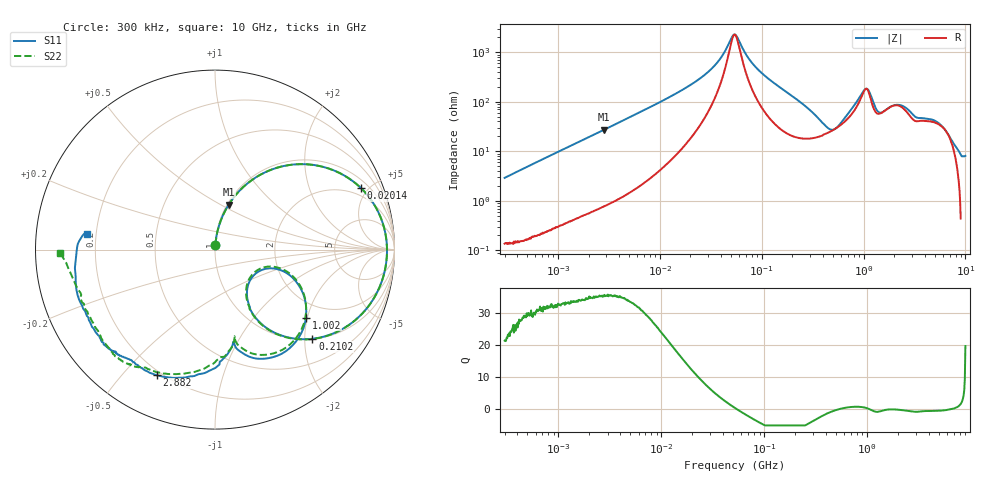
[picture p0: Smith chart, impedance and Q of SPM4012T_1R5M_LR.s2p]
! S-Parameter Data Generated by TDK Corporation
! Copyright(C) 2019 TDK Corporation.
! All Rights Reserved.
! TDK P/N: SPM4012T-1R5M-LR (Inductor)
! Property: L=1.5uH at 100kHz
! Size(LxWxT): 4.4x4.1x1.2mm
! Model Type: s2p (Touchstone File Format Version 1.0)
! Frequency: DC=Yes Start=0.3MHz Stop=10000MHz 802points Log-sweep
! Model Generated on Sep. 23, 2019
! Port Assignments:
!  1 ---@@@--- 2
! Applicable Conditions:
!  Temperature = 25 degC
!  DC Bias Current = 0 A
!  Small Signal Operation
! Terms and conditions regarding TDK Simulation Models
! (1)This simulation model is being provided solely for informational purposes. Please refer to the specifications of the products in terms of detailed characteristics of such products.
! (2)In no event shall TDK Corporation of any of its subsidiaries be liable for any loss or damage arising, directly or indirectly,
!  From any information contained in this simulation model, including, but not limited to loss or damages arising from any inaccuracies, omissions or errors in connection with such information.
! (3)Any and all copyrights on this simulation model are owned by TDK Corporation.
!  Duplication or redistribution of this simulation model without prior written permission from TDK Corporation is prohibited.
! (4)This simulation model is subject to any modification or change without any prior notice.
! (5)Neither TDK Corporation nor any of its subsidiaries shall make any warranty, express or implied,
!  Including but not limited to the correctness, implied warranties of merchantability and fitness for a particular purpose with respect to this simulation models.
! (6)The use of this simulation model shall be deemed to have consented to the terms and conditions hereof.
# Hz S MA R 50
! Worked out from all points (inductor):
!   801 points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, 300 kHz to 10 GHz, reference 50 ohm
!   read as one part in series: L = 1.55 uH near 318.3 kHz
!   highest Q = 35.3 at 2.857 MHz (marker M1), where L = 1.53 uH
!   self-resonance near 54.41 MHz
!   S11 on the Smith chart (normalised r, x): 300 kHz: 1.00, +0.06; 20.14 MHz: 1.45, +4.51; 210.2 MHz: 1.01, -2.18; 1.002 GHz: 1.55, -1.96; 2.882 GHz: 0.18, -0.62; 10 GHz: 0.17, +0.06
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300000  0.02814 85.6  0.9981 -1.7  0.9984 -1.7  0.02796 85.3
1713600  0.1618 78.9  0.9821 -9.4  0.9821 -9.4  0.1617 78.9
2857356  0.2617 73.1  0.9577 -15.3  0.9578 -15.3  0.2617 73.1
9671944  0.6725 45.1  0.713 -42.6  0.7131 -42.6  0.6724 45.1
2.013744e7  0.8828 22.8  0.4015 -62.4  0.4016 -62.4  0.8828 22.8
3.467969e7  0.9473 8.5  0.1749 -68.9  0.1749 -68.9  0.9473 8.5
5.477226e7  0.958 -2.2  0.04202 1.1  0.04203 1.1  0.9581 -2.3
9.327145e7  0.9317 -15.4  0.2115 61.8  0.2116 61.8  0.9317 -15.5
2.102074e8  0.7359 -42.5  0.5739 38.6  0.574 38.6  0.735 -42.7
3.126428e8  0.5295 -56.4  0.7247 18.8  0.7248 18.8  0.5275 -56.7
4.20949e8  0.3507 -58.0  0.7739 1.6  0.774 1.6  0.3465 -58.4
5.663179e8  0.2583 -35.1  0.7495 -17.1  0.7495 -17.1  0.2495 -34.7
7.84152e8  0.4135 -18.0  0.5965 -38.6  0.5965 -38.6  0.4051 -16.5
1.001841e9  0.6328 -36.8  0.3544 -42.8  0.3544 -42.8  0.6204 -35.3
1.180962e9  0.6802 -61.9  0.3702 -15.5  0.3702 -15.5  0.6638 -60.5
1.35547e9  0.5752 -76.9  0.4999 -23.4  0.5 -23.4  0.555 -75.8
1.767019e9  0.5623 -81.1  0.4464 -46.3  0.4464 -46.4  0.5286 -78.8
2.882439e9  0.772 -114.9  0.3385 -51.9  0.3385 -51.9  0.7493 -112.8
4.749267e9  0.8017 -135.3  0.2858 -74.1  0.2858 -74.1  0.8099 -130.2
6.091595e9  0.8078 -144.6  0.2678 -86.8  0.2681 -86.9  0.7999 -144.1
7.875699e9  0.7904 -169.1  0.2316 -109.8  0.2319 -109.9  0.805 -167.5
1e10  0.7176 172.9  0.1761 -123.7  0.1761 -123.8  0.8648 -178.7
